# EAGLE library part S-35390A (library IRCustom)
S-35390A 2-WIRE REAL-TIME CLOCK The S-35390A is a CMOS 2-wire real-time clock IC which operates with the very low current consumption and in the wide range of operation voltage. The operation voltage is 1.3 V to 5.5 V so that this IC can be used for various power supplies from main supply to backup battery. Due to the 0.25 ?A current consumption and wide range of power supply voltage at time keeping, this IC makes the battery life longer. In the system which operates with a backup battery, the included free registers can be used as the function for user?s backup memory
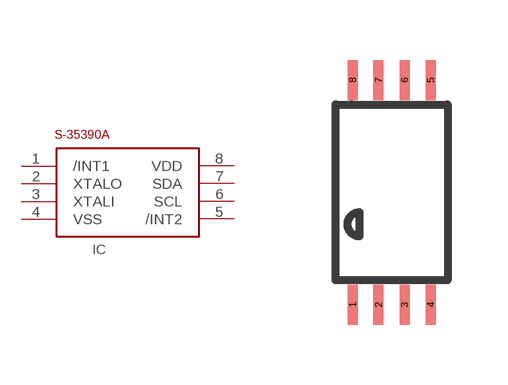
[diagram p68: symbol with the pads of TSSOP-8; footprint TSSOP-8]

Designator prefix IC

## S-35390A-T  [TSSOP-8]
1  /INT1  out
2  XTALO  out
3  XTALI  in
4  VSS  pwr
5  /INT2  out
6  SCL  in
7  SDA
8  VDD  pwr

## Footprint TSSOP-8 (pad centres in mm)
smd 0.25 x 1: 1 -0.975,-2.813; 2 -0.325,-2.813; 3 0.325,-2.813; 4 0.975,-2.813; 5 0.975,2.813; 6 0.325,2.813; 7 -0.325,2.813; 8 -0.975,2.813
